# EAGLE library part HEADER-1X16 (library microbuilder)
PIN HEADER
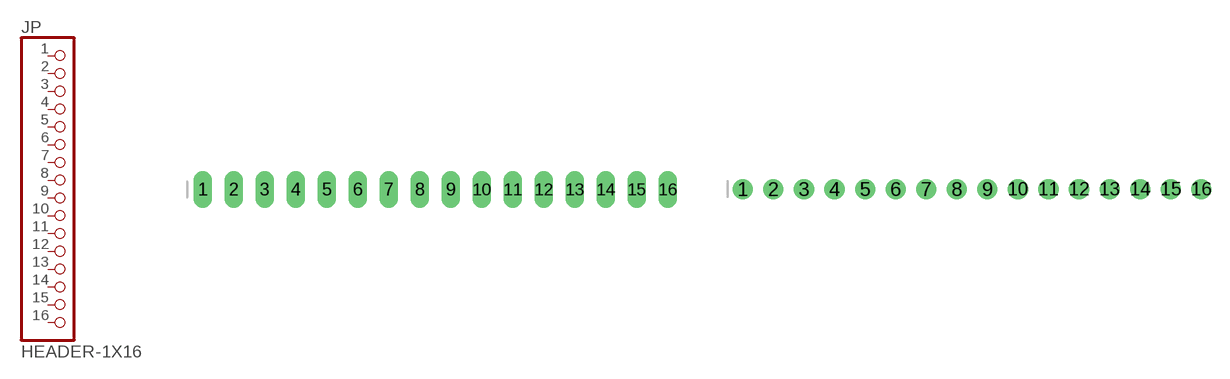
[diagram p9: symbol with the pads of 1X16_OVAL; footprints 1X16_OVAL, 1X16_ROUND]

Designator prefix JP

## HEADER-1X16  [1X16_OVAL]
1  1  pas
2  2  pas
3  3  pas
4  4  pas
5  5  pas
6  6  pas
7  7  pas
8  8  pas
9  9  pas
10  10  pas
11  11  pas
12  12  pas
13  13  pas
14  14  pas
15  15  pas
16  16  pas

## HEADER-1X16ROUND  [1X16_ROUND]
Pads as for 1X16_OVAL

## HEADER-1X162MM  [1X16_2MM]
P$1  1  pas
P$2  2  pas
P$3  3  pas
P$4  4  pas
P$5  5  pas
P$6  6  pas
P$7  7  pas
P$8  8  pas
P$9  9  pas
P$10  10  pas
P$11  11  pas
P$12  12  pas
P$13  13  pas
P$14  14  pas
P$15  15  pas
P$16  16  pas

## HEADER-1X162MM_OVAL  [1X16_2MM_OVAL]
Pads as for 1X16_2MM

## Footprint 1X16_OVAL (pad centres in mm)
PIN HEADER
drill 1 long: 1 -19.05,0; 2 -16.51,0; 3 -13.97,0; 4 -11.43,0; 5 -8.89,0; 6 -6.35,0; 7 -3.81,0; 8 -1.27,0; 9 1.27,0; 10 3.81,0; 11 6.35,0; 12 8.89,0; 13 11.43,0; 14 13.97,0; 15 16.51,0; 16 19.05,0

## Footprint 1X16_ROUND (pad centres in mm)
PIN HEADER
drill 1 pad 1.676: 1 -19.05,0; 2 -16.51,0; 3 -13.97,0; 4 -11.43,0; 5 -8.89,0; 6 -6.35,0; 7 -3.81,0; 8 -1.27,0; 9 1.27,0; 10 3.81,0; 11 6.35,0; 12 8.89,0; 13 11.43,0; 14 13.97,0; 15 16.51,0; 16 19.05,0

## Footprint 1X16_2MM (pad centres in mm)
drill 0.8 pad 1.27: P$1 -15,0; P$2 -13,0; P$3 -11,0; P$4 -9,0; P$5 -7,0; P$6 -5,0; P$7 -3,0; P$8 -1,0; P$9 1,0; P$10 3,0; P$11 5,0; P$12 7,0; P$13 9,0; P$14 11,0; P$15 13,0; P$16 15,0

## Footprint 1X16_2MM_OVAL (pad centres in mm)
drill 0.8 pad 1.27 long: P$1 -15,0; P$2 -13,0; P$3 -11,0; P$4 -9,0; P$5 -7,0; P$6 -5,0; P$7 -3,0; P$8 -1,0; P$9 1,0; P$10 3,0; P$11 5,0; P$12 7,0; P$13 9,0; P$14 11,0; P$15 13,0; P$16 15,0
